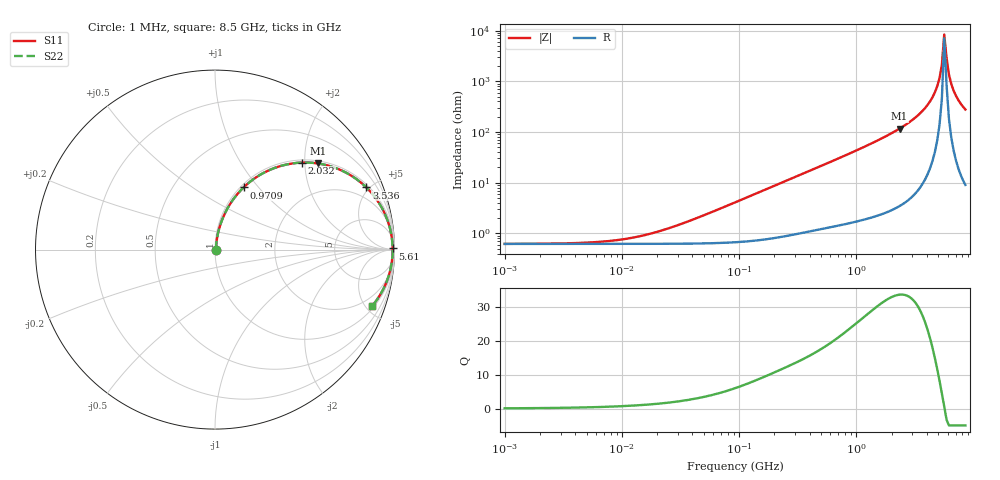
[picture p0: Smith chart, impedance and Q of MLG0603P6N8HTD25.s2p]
! S-Parameter Data Generated by TDK Corporation
! Copyright(C) 2025 TDK Corporation.
! All Rights Reserved.
! TDK P/N: MLG0603P6N8HTD25 (SMD / SMT Inductor (Coil))
! Property: L=6.8nH at 500MHz
! Size(LxWxT): 0.6x0.3x0.3mm
! Model Type: s2p (Touchstone File Format Version 1.0)
! Frequency: DC=Yes Start=1MHz Stop=8500MHz 198points Log-sweep
! Model Generated on Feb. 6, 2025
! Terms and conditions regarding TDK Simulation Models:
! 1)This simulation model is being provided solely for informational
!  purposes. Please refer to the specifications of the products in
!  terms of detailed characteristics of such products.
! 2)In no event shall TDK Corporation of any of its subsidiaries be
!  liable for any loss or damage arising, directly or indirectly,
!  from any information contained in this simulation model, including,
!  but not limited to loss or damages arising from any inaccuracies,
!  omissions or errors in connection with such information.
! 3)Any and all copyrights on this simulation model are owned by
!  TDK Corporation.  Duplication or redistribution of this simulation
!  model without prior written permission from TDK Corporation
!  is prohibited.
! 4)This simulation model is subject to any modification or change
!  without any prior notice.
! 5)Neither TDK Corporation nor any of its subsidiaries shall make any
!  warranty, express or implied, including but not limited to the
!  correctness, implied warranties of merchantability and fitness for
!  a particular purpose with respect to this simulation models.
! 6)The use of this simulation model shall be deemed to have consented
!  to the terms and conditions hereof.
! Port Assignments:
!  1 ---@@@--- 2
! Applicable Conditions:
!  Temperature = 25 degC
!  DC Bias Current = 0 A
!  Small Signal Operation
# Hz S MA R 50
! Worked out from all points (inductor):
!   197 points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, 1 MHz to 8.5 GHz, reference 50 ohm
!   read as one part in series: L = 6.96 nH near 44.05 MHz
!   highest Q = 33.7 at 2.334 GHz (marker M1), where L = 7.94 nH
!   self-resonance near 5.61 GHz
!   S11 on the Smith chart (normalised r, x): 1 MHz: 1.01, +0.00; 970.9 MHz: 1.03, +0.84; 2.032 GHz: 1.06, +1.93; 3.536 GHz: 1.17, +4.79; 5.61 GHz: open; 8.5 GHz: 1.18, -5.54
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1000000  0.006177 4.0  0.9938 -0.0  0.9938 -0.0  0.006177 4.0
4587603  0.006478 17.8  0.9938 -0.1  0.9938 -0.1  0.006478 17.8
1.053054e7  0.007682 36.3  0.9938 -0.3  0.9938 -0.3  0.007682 36.3
2.10461e7  0.01105 55.4  0.9938 -0.5  0.9938 -0.5  0.01105 55.4
9.219544e7  0.04048 78.3  0.9926 -2.3  0.9926 -2.3  0.04048 78.3
4.229561e8  0.1766 76.3  0.9734 -10.1  0.9734 -10.1  0.1766 76.3
9.708683e8  0.381 65.3  0.9094 -22.4  0.9094 -22.4  0.381 65.3
1.404574e9  0.5212 56.7  0.8359 -31.4  0.8359 -31.4  0.5212 56.7
1.940355e9  0.6641 46.7  0.7277 -41.6  0.7277 -41.6  0.6641 46.7
2.032026e9  0.6851 45.0  0.708 -43.2  0.708 -43.2  0.6851 45.0
2.333852e9  0.7479 39.9  0.642 -48.4  0.642 -48.4  0.7479 39.9
3.535948e9  0.9117 22.3  0.3804 -65.7  0.3804 -65.7  0.9117 22.3
4.253027e9  0.9599 13.7  0.2378 -73.5  0.2378 -73.5  0.9599 13.7
4.884749e9  0.9818 7.1  0.124 -78.0  0.124 -78.0  0.9818 7.1
5.115526e9  0.9861 4.9  0.08533 -78.2  0.08533 -78.2  0.9861 4.9
5.357206e9  0.9889 2.6  0.04673 -74.9  0.04673 -74.9  0.9889 2.6
5.610304e9  0.99 0.4  0.01184 -32.3  0.01184 -32.3  0.99 0.4
5.87536e9  0.9896 -1.9  0.03433 71.4  0.03433 71.4  0.9896 -1.9
6.152938e9  0.9876 -4.1  0.07275 78.1  0.07275 78.1  0.9876 -4.1
6.44363e9  0.984 -6.4  0.1116 78.6  0.1116 78.6  0.984 -6.4
7.066863e9  0.9721 -10.9  0.1885 76.1  0.1885 76.1  0.9721 -10.9
8.5e9  0.9309 -19.6  0.3361 68.5  0.3361 68.5  0.9309 -19.6
